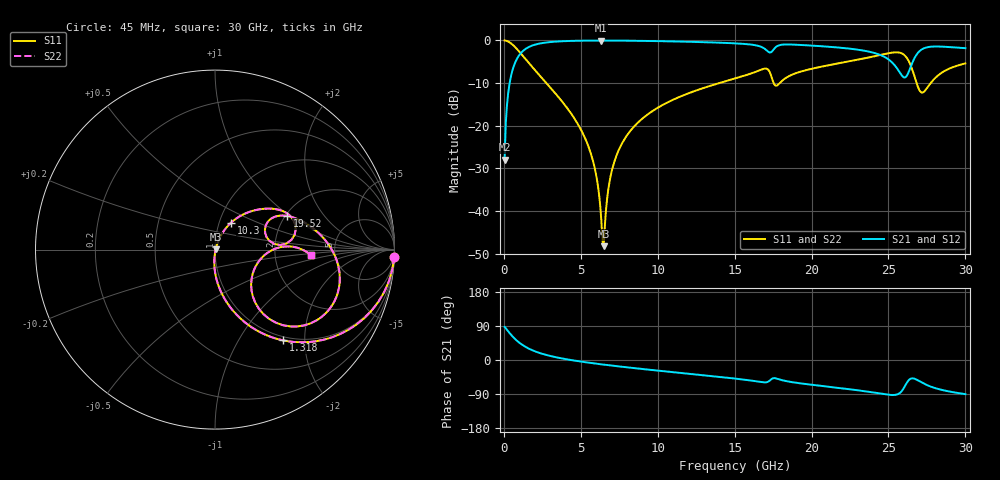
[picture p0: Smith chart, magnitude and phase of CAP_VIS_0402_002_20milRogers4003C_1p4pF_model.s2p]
! S-parameter model data by Modelithics Inc.  support@modelithics.com  813-866-6335  Tampa FL USA
! S-Parameter data specifications:
! Substrate: 20-mil Rogers 4003C, substrate thickness, H=0.508mm, Dielectric constant, Er=3.75
! PCB Mounting Pad Footprint: Pad width, PadW=0.50mm , Pad length, PadL=0.50mm , Pad gap, PadG (edge-to-edge)=0.40mm , Reference planes=1.4mm apart
! Created Wed Nov 18 12:35:28 2015
# hz S ma R 50
! 2 Port Network Data from SP1.SP block
! freq  magS11  angS11  magS21  angS21  magS12  angS12  magS22  angS22
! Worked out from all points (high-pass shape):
!   401 points, 45 MHz to 30 GHz, reference 50 ohm
!   highest |S21| = -0.03 dB at 6.336 GHz (marker M1); lowest = -27.9 dB at 45 MHz (marker M2)
!   |S21| within 3 dB of the highest: 1.088 GHz to 24.17 GHz (23.08 GHz wide, 183 % of centre); 26.89 GHz to end of sweep
!   lowest |S11| = -48.2 dB at 6.485 GHz (marker M3), VSWR 1.01, Z = 50.4 + j0.0704 ohm
!   |S11| at or under -10 dB: 2.758 GHz to 14 GHz (11.24 GHz wide, 134 % of centre); 17.54 GHz to 17.93 GHz (392.7 MHz wide, 2.21 % of centre); 26.83 GHz to 27.74 GHz (914.8 MHz wide, 3.35 % of centre)
!   |S22| runs from -48.2 to 0.0 dB; largest |S21 - S12| = 0
!   S11 on the Smith chart (normalised r, x): 45 MHz: 1, -48; 1.318 GHz: 0.94, -1.58; 10.3 GHz: 1.14, +0.35; 19.52 GHz: 2.04, +0.95; 30 GHz: 3.29, -0.30
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4.5e7  0.9992 -2.4  0.04005 87.6  0.04005 87.6  0.9992 -2.4
2.696625e8  0.9722 -14.0  0.2339 76.0  0.2339 76.0  0.9722 -14.0
4.94325e8  0.9142 -24.8  0.4048 65.2  0.4048 65.2  0.9142 -24.8
1.318088e9  0.6321 -53.1  0.7736 36.7  0.7736 36.7  0.6321 -53.1
2.666062e9  0.3302 -75.3  0.9417 14.3  0.9417 14.3  0.3302 -75.3
5.062462e9  0.08611 -92.4  0.993 -4.5  0.993 -4.5  0.08611 -92.4
5.886225e9  0.03292 -93.2  0.9959 -9.1  0.9959 -9.1  0.03292 -93.2
6.33555e9  0.007646 -73.9  0.9962 -11.4  0.9962 -11.4  0.007646 -73.9
6.485325e9  0.003879 10.4  0.9962 -12.2  0.9962 -12.2  0.003879 10.4
6.93465e9  0.02557 67.3  0.9957 -14.4  0.9957 -14.4  0.02557 67.3
7.458862e9  0.05161 68.8  0.9946 -16.9  0.9946 -16.9  0.05161 68.8
1.007992e10  0.1658 60.1  0.9812 -28.3  0.9812 -28.3  0.1658 60.1
1.030459e10  0.1747 59.2  0.9796 -29.3  0.9796 -29.3  0.1747 59.2
1.50225e10  0.358 39.5  0.9241 -49.0  0.9241 -49.0  0.358 39.5
1.74189e10  0.3635 4.0  0.7402 -49.6  0.7402 -49.6  0.3635 4.0
1.951575e10  0.4424 25.1  0.8804 -62.9  0.8804 -62.9  0.4424 25.1
2.003996e10  0.4668 22.8  0.8693 -65.5  0.8693 -65.5  0.4668 22.8
2.505742e10  0.7105 -12.0  0.5886 -91.9  0.5886 -91.9  0.7105 -12.0
2.618074e10  0.628 -43.0  0.3827 -60.9  0.3827 -60.9  0.628 -43.0
2.692961e10  0.281 -44.2  0.721 -54.0  0.721 -54.0  0.281 -44.2
2.790315e10  0.3424 1.2  0.8473 -72.5  0.8473 -72.5  0.3424 1.2
3e10  0.5375 -3.5  0.811 -90.1  0.811 -90.1  0.5375 -3.5
